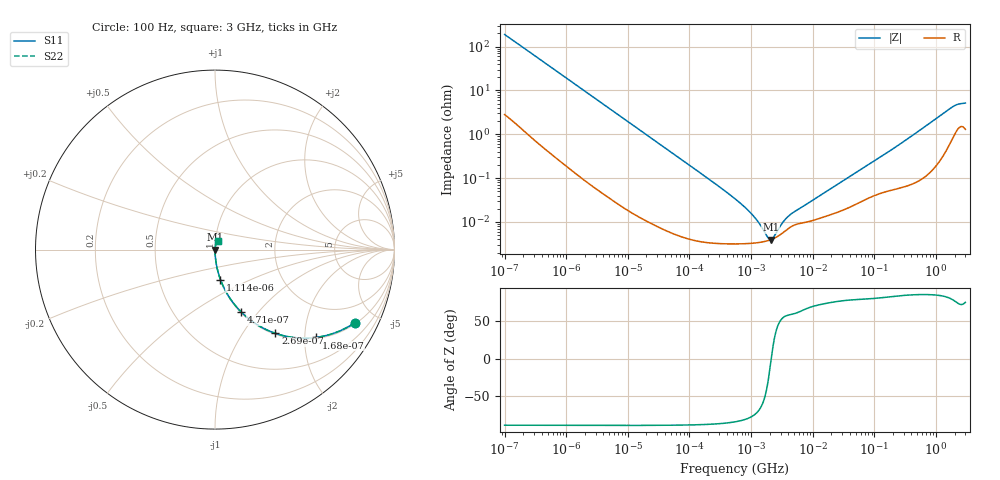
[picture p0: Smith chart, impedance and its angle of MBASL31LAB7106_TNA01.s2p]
! MBASL31LAB7106_TNA01  S-PARAMETER MODEL  ( Standard Model )
! Model Generated by TAIYO YUDEN Corporation (http://www.ty-top.com)
! Version 1.0
! TAIYO YUDEN Control No. 220601
! Copyright(c) 2012 TAIYO YUDEN CO.,LTD. All Rights Reserved.
! Product Description (link to TY-COMPAS)
! https://ds.yuden.co.jp/TYCOMPAS/or/detail?pn=MBASL31LAB7106KTNA01&u=M
! Products Name : Multilayer Ceramic Capacitors
! Characteristics :
!  Capacitance : 10 [uF] , Rated Voltage : 10 [V] , TCC : X7R
!  Case Size : 3.2 x 1.6 / 0.126 x 0.063 [mm/inch] , Thickness : 1.6 / 0.063 [mm/inch]
!  (Conditions: Temperature = 25 [degC] , DC Bias Voltage = 0 [V])
! External Node Assignments :
!  1  o---| |---o  2
! GND o---------o GND
! Frequency Range : 100Hz  -  3GHz  [ 401 STEP ]
# MHZ S RI R 50
! Freq[MHz].  S11 Real  S11 Imag  S21 Real  S21 Imag  S12 Real  S12 Imag  S22 Real  S22 Imag
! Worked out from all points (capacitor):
!   401 points, 100 Hz to 3 GHz, reference 50 ohm
!   read as one part in series: C = 8.39 uF near 109 Hz
!   lowest |Z| = 3.95 mohm at 2.08 MHz (marker M1)
!   series resonance near 2.121 MHz, so ESL is about 670 pH
!   S11 on the Smith chart (normalised r, x): 100 Hz: 1.06, -3.78; 168 Hz: 1.03, -2.27; 269 Hz: 1.02, -1.42; 471 Hz: 1.01, -0.81; 1.114 kHz: 1.00, -0.35; 3 GHz: 1.03, +0.10
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0.0001  0.7779 -0.4083  0.2221 0.4083  0.2221 0.4083  0.7779 -0.4083
0.000168  0.5618 -0.4894  0.4382 0.4894  0.4382 0.4894  0.5618 -0.4894
0.000269  0.3365 -0.4665  0.6635 0.4665  0.6635 0.4665  0.3365 -0.4665
0.000471  0.1446 -0.3464  0.8554 0.3464  0.8554 0.3464  0.1446 -0.3464
0.000694  0.0734 -0.2557  0.9266 0.2557  0.9266 0.2557  0.0734 -0.2557
0.001114  0.0305 -0.1673  0.9695 0.1673  0.9695 0.1673  0.0305 -0.1673
0.001788  0.0125 -0.1065  0.9875 0.1065  0.9875 0.1065  0.0125 -0.1065
0.005476  0.00157 -0.0354  0.9984 0.0354  0.9984 0.0354  0.00157 -0.0354
0.031977  0.000112 -0.00612  0.9999 0.00612  0.9999 0.00612  0.000112 -0.00612
0.221826  3.38e-05 -0.00088  1 0.00088  1 0.00088  3.38e-05 -0.00088
0.547723  3.16e-05 -0.000336  1 0.000336  1 0.000336  3.16e-05 -0.000336
0.842342  3.2e-05 -0.000197  1 0.000197  1 0.000197  3.2e-05 -0.000197
1.295438  3.37e-05 -9.56e-05  1 9.56e-05  1 9.56e-05  3.37e-05 -9.56e-05
1.411895  3.43e-05 -7.79e-05  1 7.79e-05  1 7.79e-05  3.43e-05 -7.79e-05
2.079876  3.93e-05 -3.57e-06  1 3.57e-06  1 3.57e-06  3.93e-05 -3.57e-06
3.198641  5.52e-05 7.58e-05  0.9999 -7.58e-05  0.9999 -7.58e-05  5.52e-05 7.58e-05
4.711951  8.14e-05 0.000139  0.9999 -0.000139  0.9999 -0.000139  8.14e-05 0.000139
9.794414  0.000107 0.00029  0.9999 -0.00029  0.9999 -0.00029  0.000107 0.00029
175.1444  0.000531 0.00407  0.9995 -0.00407  0.9995 -0.00407  0.000531 0.00407
1789.813  0.00875 0.0395  0.9912 -0.0395  0.9912 -0.0395  0.00875 0.0395
2219.584  0.0145 0.045  0.9855 -0.045  0.9855 -0.045  0.0145 0.045
3000  0.0152 0.0487  0.9848 -0.0487  0.9848 -0.0487  0.0152 0.0487
